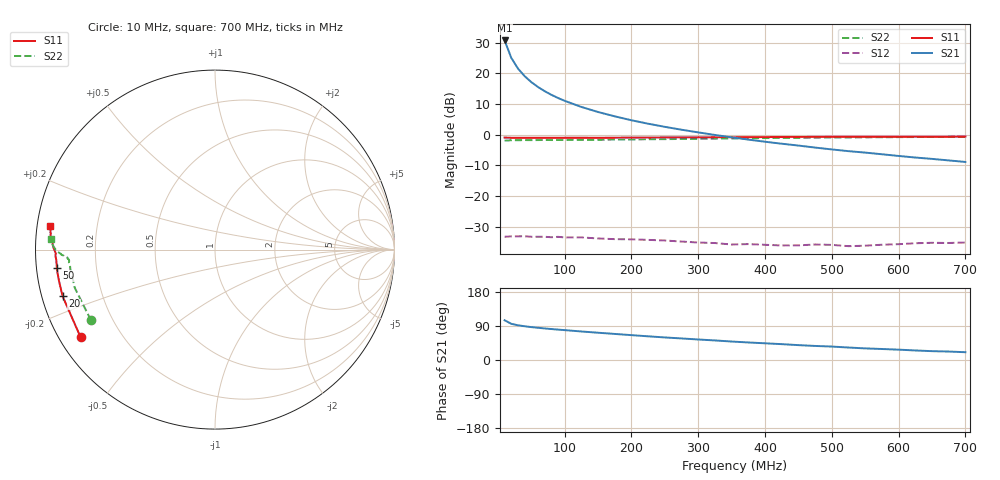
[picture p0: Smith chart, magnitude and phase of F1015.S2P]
! Date: Mon Aug 07 16:40:39 1995
# MHZ  S  MA  R  50.0000
!  POLYFET RF DEVICES
!  F1015
!  S PARAMETERS
!  VDS=28V, IDQ=800mA
!FREQ  S11MAG S11ANG S21MAG S21ANG S12MAG S12ANG S22MAG S22ANG
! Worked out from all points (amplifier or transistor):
!   34 points, 10 MHz to 700 MHz, reference 50 ohm
!   highest |S21| = 30.7 dB at 10 MHz (marker M1)
!   |S21| within 3 dB of that: start of sweep to 15.29 MHz
!   unconditionally stable (mu >= 1): 327.3 MHz to end of sweep
!   at 60 MHz: K = 0.15, MSG = 24.4 dB, |S12| = -33.3 dB
!   at 300 MHz: K = 0.86, MSG = 17.9 dB, |S12| = -35.2 dB
!   at 700 MHz: K = 1.52, MAG = 8.9 dB, |S12| = -35.2 dB
!   S11 on the Smith chart (normalised r, x): 10 MHz: 0.06, -0.30; 20 MHz: 0.06, -0.15; 50 MHz: 0.06, -0.06; 700 MHz: 0.04, +0.07
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10  0.8942 -146.8  34.21 104.8  0.02161 15.6  0.7956 -150.3
20  0.888 -163.0  17.8 95.5  0.02195 8.6  0.8098 -164.7
30  0.8865 -168.7  11.92 91.6  0.022 4.3  0.809 -169.5
40  0.887 -171.6  8.957 89.0  0.02205 5.1  0.8134 -172.1
50  0.8871 -173.4  7.161 86.8  0.02162 2.7  0.8127 -173.4
60  0.886 -174.7  5.959 85.0  0.02163 0.5  0.8138 -174.2
70  0.8864 -175.4  5.102 83.2  0.02161 1.1  0.8172 -175.0
80  0.8859 -176.1  4.452 81.7  0.02125 1.2  0.8146 -175.6
90  0.8872 -176.8  3.946 80.2  0.02156 0.6  0.8155 -175.9
100  0.8888 -177.3  3.549 78.8  0.02109 -0.7  0.8152 -176.0
125  0.8894 -178.0  2.821 75.3  0.0211 -1.2  0.823 -176.5
150  0.887 -178.6  2.333 72.0  0.02029 -2.1  0.8233 -176.9
175  0.8911 -179.3  1.983 68.8  0.01977 -1.5  0.8292 -177.2
200  0.894 -179.8  1.711 65.6  0.01963 -1.2  0.8315 -177.3
225  0.8955 179.9  1.504 62.5  0.01923 -0.0  0.8411 -177.5
250  0.8989 179.6  1.338 59.5  0.0188 -0.6  0.843 -177.6
300  0.9028 178.8  1.086 54.1  0.01742 1.0  0.8564 -178.1
375  0.9083 177.2  0.8285 46.3  0.01642 9.0  0.8702 -178.9
475  0.9178 175.6  0.6143 37.1  0.01618 15.3  0.8899 179.7
525  0.9197 174.8  0.537 32.9  0.01519 23.3  0.8991 179.0
600  0.9218 173.6  0.4486 27.3  0.01637 33.2  0.909 177.9
700  0.9282 171.7  0.3583 20.5  0.01742 41.5  0.9178 176.4
